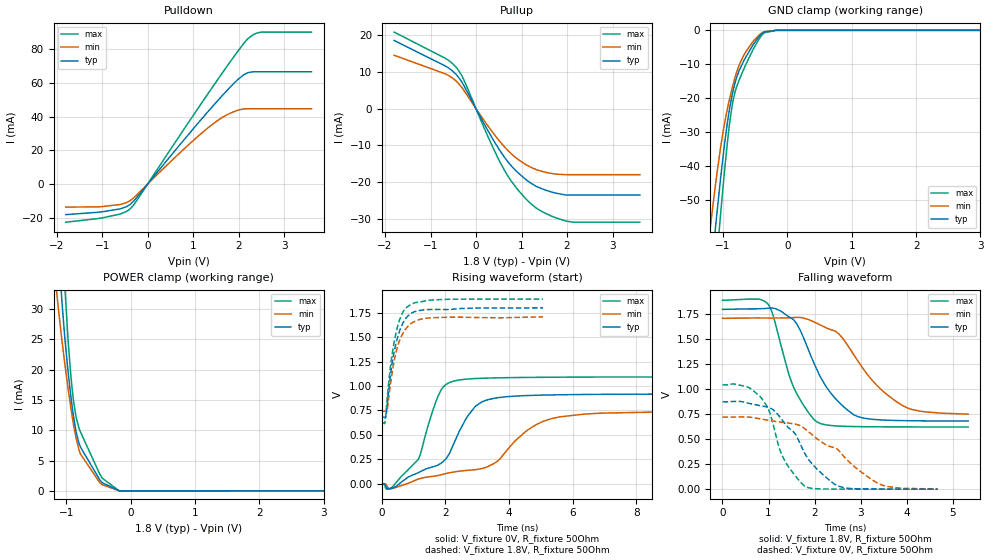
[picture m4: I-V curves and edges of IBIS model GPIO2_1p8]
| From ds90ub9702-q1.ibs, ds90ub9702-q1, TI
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|   GPIO2_1p8 Model
[Model]   GPIO2_1p8
Model_type   I/O
Polarity   Non-Inverting
Enable   Active-Low
Vinl = 0.63
Vinh = 1.17
Vmeas = 0.9
Vref = 0
Cref = 2pF
Rref = 80
|   typ   min   max
|   (nom PVT)   (fast PVT)   (slow PVT)
C_comp   5.632e-13   5.615e-13   5.751e-13
| Where nom  PVT is Nominal Process, 1.8V, 27C
|   Fast PVT is Strong Process,  1.89V, -40C
|   Slow PVT is Weak Process,   1.71V, 125C
[Voltage Range]   1.8   1.71   1.89
|Junction Temperature
[Temperature Range]   27   125   -40
[Pullup Reference]   1.8   1.71   1.89
[Pulldown Reference]   0   0   0
[Power Clamp Reference]   1.8   1.71   1.89
[GND Clamp Reference]   0   0   0
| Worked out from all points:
|   slope of the pulldown table from 0 to 0.27 V, typ, clamps not added: 30.2 ohm
|   slope of the pullup table from 0 to 0.27 V, typ, clamps not added: 43.9 ohm
|   GND clamp passes 1 mA (typ) near -0.40 V on its own axis
|   falling waveform, V_fixture 1.8V, R_fixture 50Ohm: 20-80 % time 754ps typ, 991ps min, 552ps max; typ from 1.8 V to 0.682 V
|   rising waveform, V_fixture 0V, R_fixture 50Ohm: 20-80 % time 1.09ns typ, 1.77ns min, 670ps max; typ from 0 V to 0.874 V
|   rising waveform, V_fixture 1.8V, R_fixture 50Ohm: 20-80 % time 375ps typ, 386ps min, 350ps max; typ from 0.681 V to 1.8 V
|   falling waveform, V_fixture 0V, R_fixture 50Ohm: 20-80 % time 828ps typ, 1.23ns min, 501ps max; typ from 0.875 V to 0 V
[Pulldown]
|   Voltage   I(typ)   I(min)   I(max)
-1.8V     -18.1mA    -13.63mA   -22.58mA
-1.118V   -16.75mA   -13.52mA   -20.52mA
-616.7mV  -14.76mA   -12.15mA   -17.83mA
-370.8mV  -11.74mA   -9.517mA   -14.31mA
682.9mV   22.51mA    17.91mA    27.88mA
1.375V    44.46mA    34.38mA    55.51mA
1.806V    57.22mA    41.87mA    72.16mA
2.108V    64.69mA    44.51mA    83.23mA
2.222V    66.11mA    44.62mA    86.57mA
2.351V    66.54mA    44.62mA    88.92mA
2.507V    66.54mA    44.62mA    90.02mA
3.6V      66.54mA    44.62mA    90.04mA
[GND Clamp]
|   Voltage   I(typ)   I(min)   I(max)
-1.8V     -199mA     -165.6mA   -233.3mA
-1.222V   -78.4mA    -62.06mA   -95.77mA
-1.143V   -63.11mA   -49.48mA   -77.71mA
-1.089V   -52.94mA   -41.47mA   -65.54mA
-1.037V   -43.49mA   -34.4mA    -54.01mA
-916.2mV  -25.22mA   -21.72mA   -30.32mA
-860.4mV  -19.3mA    -17.23mA   -22.44mA
-818.5mV  -15.84mA   -14.25mA   -18.54mA
-677.3mV  -9.004mA   -7.336mA   -11.44mA
-401.4mV  -1.038mA   -808.5uA   -1.512mA
-180mV    -2.202uA   -5.833uA   -1.169uA
3.6V      0A         0A         0A
[Pullup]
|   Voltage   I(typ)   I(min)   I(max)
-1.8V     18.57mA    14.55mA    20.87mA
-687.6mV  11.7mA     9.532mA    13.79mA
-427.9mV  9.197mA    7.405mA    11.15mA
-295.6mV  6.918mA    5.493mA    8.587mA
252mV     -5.809mA   -4.572mA   -7.364mA
467.5mV   -10.33mA   -8.117mA   -13.11mA
628.7mV   -13.33mA   -10.48mA   -16.92mA
951.8mV   -17.82mA   -14.11mA   -22.6mA
1.319V    -21.16mA   -16.61mA   -27.08mA
1.761V    -23.08mA   -17.88mA   -29.82mA
2.117V    -23.57mA   -18.03mA   -30.96mA
3.6V      -23.57mA   -18.03mA   -30.98mA
[POWER Clamp]
|   Voltage   I(typ)   I(min)   I(max)
-1.8V     198.5mA    148.8mA    248.5mA
-1.154V   45.97mA    33.08mA    64.86mA
-1.133V   42mA       30.88mA    59.49mA
-1.076V   32.34mA    25.47mA    45.53mA
-1.018V   24.39mA    20.39mA    32.58mA
-930.6mV  15.62mA    13.69mA    19.01mA
-889mV    12.28mA    10.92mA    14.86mA
-849.6mV  9.778mA    8.71mA     12.16mA
-783.2mV  7.265mA    6.119mA    9.77mA
-443mV    1.358mA    1.022mA    2.099mA
-170.8mV  13.67uA    22.3uA     18.78uA
3.6V      0A         0A         0A
[Ramp]
R_load = 50
|   typ   min   max
dV/dt_r   0.524216/1.08971e-09   0.433969/1.76763e-09   0.626663/6.63653e-10
dV/dt_f   0.671531/7.55111e-10   0.580735/1.00268e-09   0.760624/5.5113e-10
[Falling Waveform]
V_fixture = 1.8V
V_fixture_min = 1.71V
V_fixture_max = 1.89V
R_fixture = 50Ohm
|   Time   V(typ)   V(min)   V(max)
0s        1.8V       1.71V      1.89V
989.9ps   1.811V     1.713V     1.853V
1.105ns   1.812V     1.713V     1.729V
1.539ns   1.697V     1.718V     1.027V
2.043ns   1.203V     1.662V     676.3mV
2.522ns   873.1mV    1.557V     631.8mV
2.928ns   728.1mV    1.29V      626.3mV
3.354ns   696.1mV    1.038V     624.3mV
3.898ns   686.4mV    839.7mV    623.2mV
5.332ns   681.7mV    750.8mV    622.5mV
[Rising Waveform]
V_fixture = 0V
V_fixture_min = 0V
V_fixture_max = 0V
R_fixture = 50Ohm
|   Time   V(typ)   V(min)   V(max)
0s        1.137uV    5.772uV    563.7nV
278.7ps   -52.12mV   -44.98mV   -47.12mV
1.136ns   111.6mV    46.77mV    245.5mV
1.695ns   182mV      80.02mV    835.8mV
2.022ns   256.9mV    104.7mV    1.017V
2.984ns   803mV      145.8mV    1.077V
4.622ns   903.1mV    557.6mV    1.088V
6.756ns   914.4mV    720.2mV    1.092V
15.43ns   920.2mV    750.7mV    1.092V
300ns     873.7mV    723.3mV    1.044V
[Rising Waveform]
V_fixture = 1.8V
V_fixture_min = 1.71V
V_fixture_max = 1.89V
R_fixture = 50Ohm
|   Time   V(typ)   V(min)   V(max)
0s        680.7mV    742.1mV    622.2mV
95.04ps   675.8mV    742.1mV    622.8mV
133.3ps   698.2mV    736.8mV    740.4mV
165.2ps   797.5mV    753.2mV    867.7mV
300.7ps   1.185V     1.084V     1.275V
458.5ps   1.454V     1.361V     1.562V
615ps     1.611V     1.51V      1.726V
812.4ps   1.714V     1.608V     1.813V
1.536ns   1.783V     1.699V     1.88V
5.068ns   1.799V     1.708V     1.89V
[Falling Waveform]
V_fixture = 0V
V_fixture_min = 0V
V_fixture_max = 0V
R_fixture = 50Ohm
|   Time   V(typ)   V(min)   V(max)
0s        874.5mV    720.8mV    1.045V
536.7ps   864mV      722.1mV    1.025V
819.8ps   836.2mV    704.4mV    926mV
1.009ns   816.4mV    688.4mV    788mV
1.306ns   686.1mV    669.1mV    326.2mV
1.584ns   549.5mV    650.3mV    132.1mV
1.816ns   334.2mV    594.6mV    22.2mV
2.629ns   15.65mV    330.5mV    721.6uV
3.446ns   841.2uV    43.68mV    240.5uV
4.667ns   172.9uV    1.062mV    93.02uV
